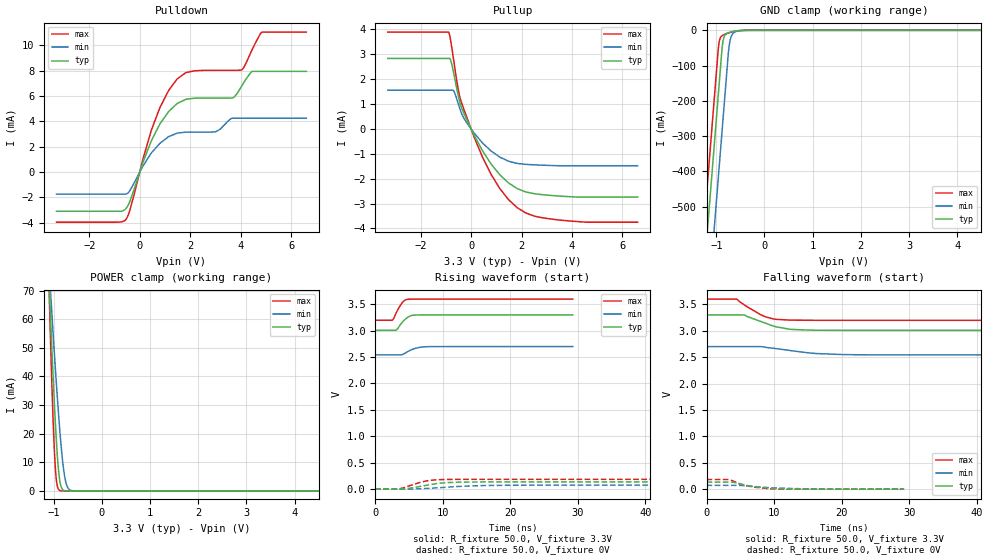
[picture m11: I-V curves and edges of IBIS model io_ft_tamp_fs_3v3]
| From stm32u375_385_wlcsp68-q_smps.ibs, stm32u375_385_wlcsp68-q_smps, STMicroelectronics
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[Model]   io_ft_tamp_fs_3v3
Model_type I/O
Polarity   Non-Inverting
Enable   Active-Low
| CAP_THRESHOLD on pad IOFT is "UDTCAPC" :
| Rising=30.0% of vddios   Falling=70.0% of vddios
| C_comp min and max val. don't necessarily correlate with the min and max pvt
| but are the smallest and greatest pad capacitance found.
| var   typ   min   max
C_comp   2.94735pF  2.92643pF  3.00916pF
|C_comp_pullup   1.82365pF  1.69752pF  1.79003pF
|C_comp_pulldown   1.12370pF  1.22891pF  1.21913pF
Vinl = 1.35V
Vinh = 1.8V
Vmeas = 1.65V   | Reference voltage for timing measurements
Cref  = 50.0pF   | Timing specification test load capacitance value
Rref  = 1.0MOhm   | Timing specification test load resistance value
Vref  = 1.815V   | Timing specification test load voltage
[Model Spec]
| TIME_THRESHOLD on pin ZIV11 is "CMOS" :
| Rising=50.0% of vdd   Falling=50.0% of vdd
Vinl 1.27950V 1.06950V 1.36550V
Vinh 1.78950V 1.51350V 1.89450V
| variable   typ   min   max
[Temperature Range] 25.0 130.0 -40.0
| variable   typ   min   max
[Voltage Range] 3.3V 2.7V 3.6V
| variable   typ   min   max
[POWER Clamp Reference] 3.3V 2.7V 3.6V
| variable   typ   min   max
[GND Clamp Reference] 0V 0V 0V
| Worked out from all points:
|   slope of the pulldown table from 0 to 0.495 V, typ, clamps not added: 190 ohm
|   slope of the pullup table from 0 to 0.495 V, typ, clamps not added: 524 ohm
|   GND clamp passes 1 mA (typ) near -0.53 V on its own axis
|   POWER clamp passes 1 mA (typ) near -0.83 V on its own axis
|   rising waveform, R_fixture 50.0, V_fixture 3.3V: 20-80 % time 1.22ns typ, 1.62ns min, 1.04ns max; typ from 3.01 V to 3.3 V
|   falling waveform, R_fixture 50.0, V_fixture 3.3V: 20-80 % time 4.07ns typ, 5.89ns min, 3.21ns max; typ from 3.3 V to 3.01 V
|   rising waveform, R_fixture 50.0, V_fixture 0V: 20-80 % time 3.73ns typ, 6.13ns min, 2.82ns max; typ from 0 V to 0.134 V
|   falling waveform, R_fixture 50.0, V_fixture 0V: 20-80 % time 3.88ns typ, 5.88ns min, 3.12ns max; typ from 0.134 V to 0 V
[POWER Clamp]
-3.3V     1.126A     769.5mA    1.647A
-1.1V     75.38mA    79.63mA    73.18mA
-1.09V    71.2mA     76.8mA     67.14mA
-1.08V    67.05mA    73.98mA    61.2mA
-1.06V    58.89mA    68.38mA    49.67mA
-1.01V    39.47mA    54.71mA    24.03mA
-970mV    25.49mA    44.18mA    9.257mA
-930mV    13.81mA    34.16mA    2.168mA
-870mV    3.251mA    20.56mA    140.6uA
-760mV    67.19uA    3.98mA     739.7nA
-630mV    518.2nA    149.1uA    1.746nA
6.6V      0A         0A         0A
[GND Clamp]
-3.3V     -4.165A    -4.4A      -4.034A
-1.25V    -679.9mA   -915.1mA   -549mA
-960mV    -186.9mA   -422.1mA   -55.97mA
-950mV    -169.9mA   -405.1mA   -42.45mA
-920mV    -118.9mA   -354.1mA   -22.92mA
-880mV    -51.66mA   -286.1mA   -15.35mA
-860mV    -30.97mA   -252.1mA   -13.65mA
-760mV    -7.32mA    -82.07mA   -8.144mA
-730mV    -5.898mA   -41.75mA   -6.789mA
-680mV    -4.176mA   -14.72mA   -4.769mA
-480mV    -457.9uA   -835.7uA   -334.7uA
6.6V      1.896nA    294.7nA    697.8pA
| variable   typ   min   max
[Pullup Reference] 3.3V 2.7V 3.6V
| variable   typ   min   max
[Pulldown Reference] 0V 0V 0V
[Pullup]
-3.3V     2.834mA    1.557mA    3.893mA
-890mV    2.834mA    1.557mA    3.893mA
-810mV    2.768mA    1.557mA    3.558mA
-690mV    2.254mA    1.529mA    2.77mA
-450mV    1.091mA    831.4uA    1.305mA
120mV     -252.2uA   -163.5uA   -324.6uA
800mV     -1.419mA   -890.9uA   -1.837mA
1.14V     -1.842mA   -1.132mA   -2.397mA
1.83V     -2.397mA   -1.387mA   -3.165mA
2.51V     -2.601mA   -1.443mA   -3.501mA
3.3V      -2.682mA   -1.473mA   -3.636mA
6.6V      -2.737mA   -1.478mA   -3.747mA
[Pulldown]
-3.3V     -3.112mA   -1.746mA   -3.972mA
-560mV    -2.917mA   -1.746mA   -3.78mA
-390mV    -2.313mA   -1.474mA   -2.998mA
460mV     2.475mA    1.504mA    3.307mA
800mV     3.8mA      2.27mA     5.099mA
1.48V     5.408mA    3.066mA    7.346mA
3.01V     5.836mA    3.17mA     8.031mA
3.67V     5.851mA    4.245mA    8.032mA
4.03V     6.763mA    4.245mA    8.067mA
4.43V     7.913mA    4.245mA    9.564mA
4.84V     7.948mA    4.245mA    11.05mA
6.6V      7.948mA    4.245mA    11.05mA
[Ramp]
dV/dt_r 80.15075mV/3.71549ns 43.44419mV/5.87691ns 109.51913mV/2.82292ns
dV/dt_f 175.11868mV/3.97581ns 94.57086mV/5.8438ns 240.9849mV/3.21151ns
R_load = 50.0
| Removed startup time: 0s 0s 0s  .
| Removed end time: 29.25ns.
[Rising Waveform]
R_fixture   = 50.0
V_fixture   = 3.3V
V_fixture_min = 2.7V
V_fixture_max = 3.6V
0s        3.008V     2.542V     3.198V
2.55ns    3.008V     2.542V     3.202V
3.15ns    3.017V     2.542V     3.353V
3.9ns     3.146V     2.544V     3.516V
4.35ns    3.207V     2.57V      3.576V
4.8ns     3.254V     2.604V     3.595V
5.5ns     3.292V     2.647V     3.598V
6.6ns     3.299V     2.685V     3.599V
7.75ns    3.299V     2.698V     3.6V
29.25ns   3.3V       2.7V       3.6V
| Removed startup time: 0s 0s 0s  .
| Removed end time: 199.25ns.
[Falling Waveform]
R_fixture   = 50.0
V_fixture   = 3.3V
V_fixture_min = 2.7V
V_fixture_max = 3.6V
0s        3.3V       2.7V       3.6V
4.45ns    3.301V     2.7V       3.598V
5.65ns    3.296V     2.7V       3.485V
7.8ns     3.186V     2.7V       3.32V
8.55ns    3.153V     2.691V     3.274V
10.1ns    3.083V     2.665V     3.22V
12.65ns   3.026V     2.621V     3.202V
16.25ns   3.011V     2.569V     3.199V
25.7ns    3.008V     2.543V     3.198V
199.3ns   3.008V     2.542V     3.198V
| Removed startup time: 0s 0s 0s  .
| Removed end time: 199.2ns.
[Rising Waveform]
R_fixture   = 50.0
V_fixture   = 0V
V_fixture_min = 0V
V_fixture_max = 0V
0s        42.36nV    238.8nV    101.2nV
3.25ns    -2.506mV   22.85uV    -2.336mV
4.1ns     -1.385mV   -1.325mV   19.3mV
5ns       11.63mV    -1.698mV   58.29mV
7.8ns     74.66mV    11.33mV    156.5mV
9.7ns     110.7mV    25.59mV    176.7mV
12.2ns    128.2mV    46.29mV    181.7mV
16.25ns   133.1mV    65.37mV    182.5mV
24.4ns    133.6mV    71.99mV    182.5mV
199.2ns   133.6mV    72.41mV    182.5mV
| Removed startup time: 0s 0s 0s  .
| Removed end time: 29.25ns.
[Falling Waveform]
R_fixture   = 50.0
V_fixture   = 0V
V_fixture_min = 0V
V_fixture_max = 0V
0s        133.6mV    72.41mV    182.5mV
3.2ns     133.6mV    72.41mV    182mV
3.95ns    129.1mV    72.39mV    154.2mV
5ns       100.3mV    70.88mV    92.68mV
5.95ns    69.84mV    61.42mV    63.13mV
7.75ns    37.68mV    42.63mV    27.92mV
10.15ns   13.57mV    23.79mV    2.804mV
12.55ns   1.268mV    13.03mV    273.9uV
17.35ns   103uV      1.143mV    27.93uV
29.25ns   1.505uV    25.6uV     239.4nV
